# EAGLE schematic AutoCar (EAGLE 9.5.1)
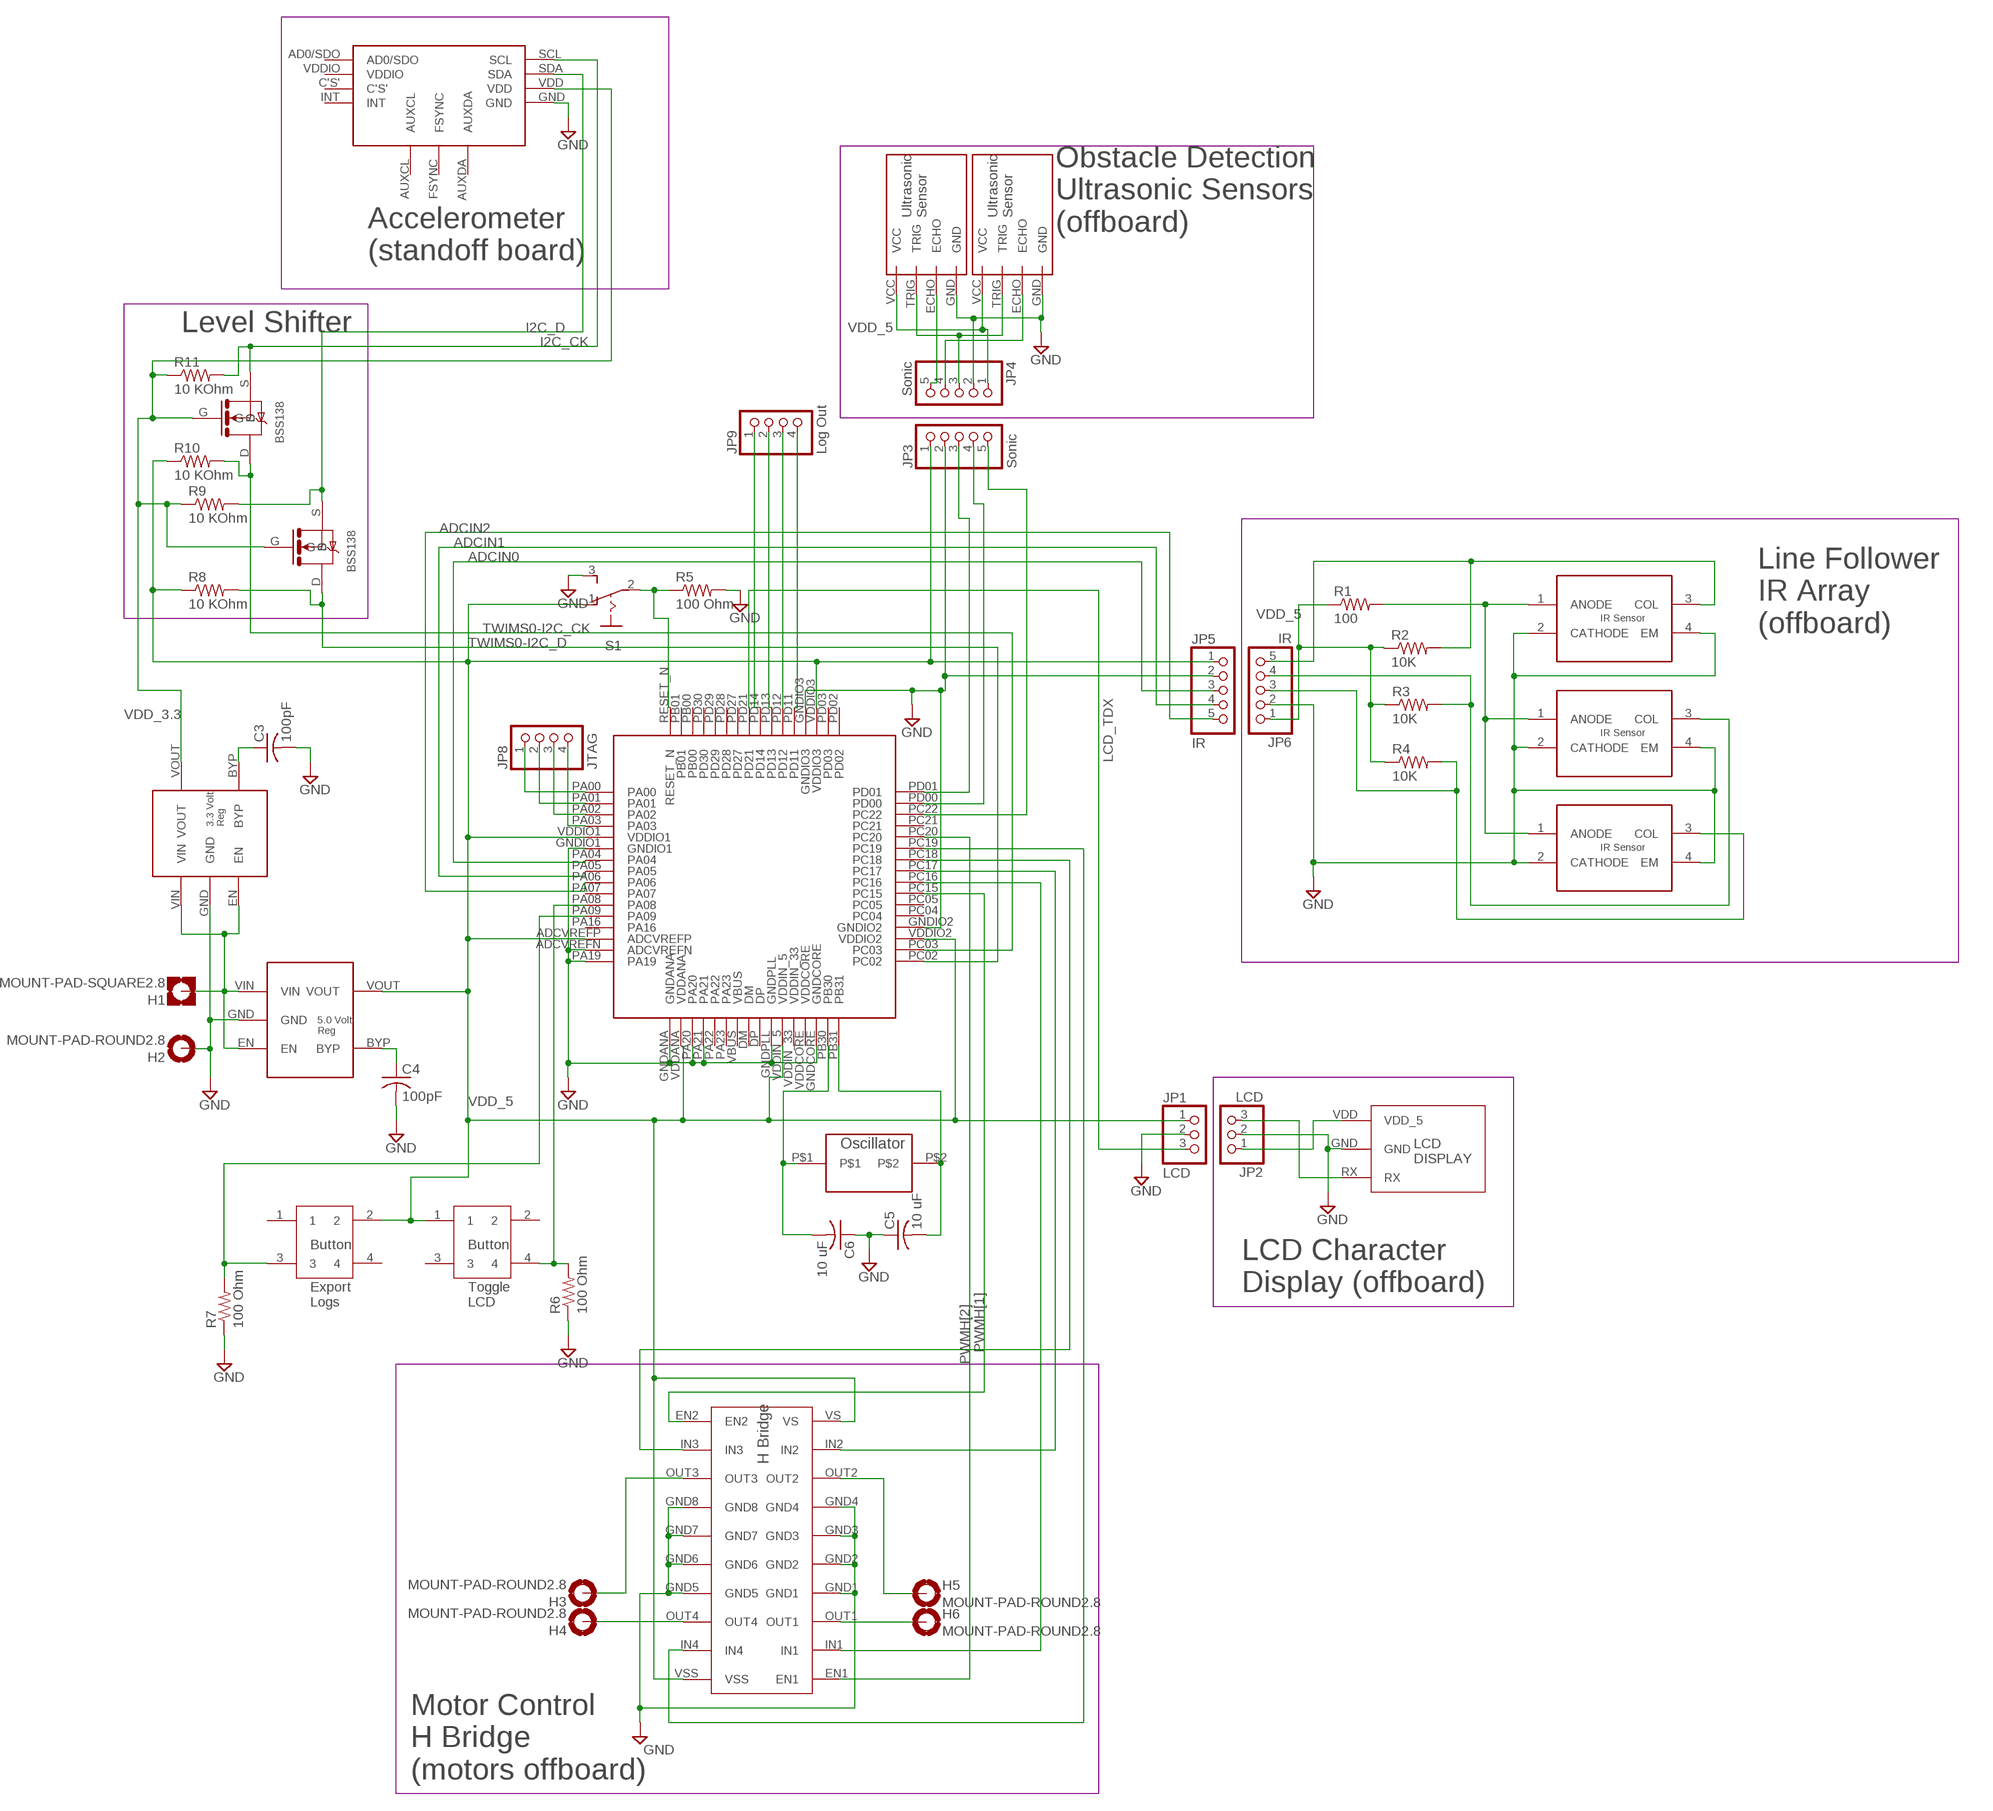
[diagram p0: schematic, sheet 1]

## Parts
C3  100pF  C-USC0805  [C0805]
C4  100pF  C-USC0805  [C0805]
C5  10 uF  C-USC0805  [C0805]
C6  10 uF  C-USC0805  [C0805]
H1  MOUNT-PAD-SQUARE2.8  [2,8-PAD-SQUARE]
H2  MOUNT-PAD-ROUND2.8  [2,8-PAD]
H3  MOUNT-PAD-ROUND2.8  [2,8-PAD]
H4  MOUNT-PAD-ROUND2.8  [2,8-PAD]
H5  MOUNT-PAD-ROUND2.8  [2,8-PAD]
H6  MOUNT-PAD-ROUND2.8  [2,8-PAD]
JP1  LCD  PINHD-1X3  [1X03]
JP2  LCD  PINHD-1X3  [1X03]
JP3  Sonic  PINHD-1X5  [1X05]
JP4  Sonic  PINHD-1X5  [1X05]
JP5  IR  PINHD-1X5  [1X05]
JP6  IR  PINHD-1X5  [1X05]
JP8  JTAG  PINHD-1X4  [1X04]
JP9  Log Out  PINHD-1X4  [1X04]
R1  100  R-US_M0805  [M0805]
R2  10K  R-US_M0805  [M0805]
R3  10K  R-US_M0805  [M0805]
R4  10K  R-US_M0805  [M0805]
R5  100 Ohm  R-US_M0805  [M0805]
R6  100 Ohm  R-US_M0805  [M0805]
R7  100 Ohm  R-US_M0805  [M0805]
R8  10 KOhm  R-US_M0805  [M0805]
R9  10 KOhm  R-US_M0805  [M0805]
R10  10 KOhm  R-US_M0805  [M0805]
R11  10 KOhm  R-US_M0805  [M0805]
S1  255SB  [255SB]
U$1  AT32UC3C2512C-A2UT  [TQFP-64]
U$2  QRE1113GR  [4-SMD]
U$3  QRE1113GR  [4-SMD]
U$4  QRE1113GR  [4-SMD]
U$5  SEN-15569  [HC-SR04]
U$6  SEN-15569  [HC-SR04]
U$7  AP2210K-5.0TRG1  [SC-74A]
U$8  SEN-13762  [MPU-9250]
U$10  AP2210K-3.3TRG1  [SC-74A]
U$11  ADAFRUIT-782  [LCD-3]
U$12  L293DD  [SOIC20]
U$14  LFXTAL003210BULK  [HC-49/US]
U$17  PTS645SM43SMTR92LFS  [SM43SMTR92LFS]
U$18  PTS645SM43SMTR92LFS  [SM43SMTR92LFS]
U$19  BSS138  [SOT23]
U$20  BSS138  [SOT23]

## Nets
ADCIN0: JP5.3 U$1.PA04
ADCIN1: JP5.4 U$1.PA05
ADCIN2: JP5.5 U$1.PA06
ECHO_L: JP3.5 JP4.5 U$1.PC22 U$6.ECHO
ECHO_R: JP3.4 JP4.4 U$1.PD00 U$5.ECHO
GND: C3.2 C4.2 C5.1 C6.1 H2.B2,8(MOUNT) JP1.2 JP2.2 JP3.2 JP4.2 JP5.2 JP6.2 R5.2 R6.1 R7.1 S1.3(S) U$1.ADCVREFN U$1.GNDANA U$1.GNDCORE U$1.GNDIO1 U$1.GNDIO2 U$1.GNDIO3 U$1.GNDPLL U$1.PA19 U$1.PA20 U$1.PA21 U$2.2(CATHODE) U$2.4(EM) U$3.2(CATHODE) U$3.4(EM) U$4.2(CATHODE) U$4.4(EM) U$5.GND U$6.GND U$7.GND U$8.GND U$10.GND U$11.GND U$12.GND1 U$12.GND2 U$12.GND3 U$12.GND4 U$12.GND5 U$12.GND6 U$12.GND7 U$12.GND8
I2C_CK: R11.2 U$8.SCL U$19.S
I2C_D: R9.2 U$8.SDA U$20.S
LCD_TDX: JP1.3 JP2.3 U$1.PD21 U$11.RX
N$1: JP2.1 U$11.VDD(VDD_5)
N$2: H3.B2,8(MOUNT) U$12.OUT3
N$3: H1.B2,8(MOUNT) U$7.EN U$7.VIN U$10.EN U$10.VIN
N$4: H4.B2,8(MOUNT) U$12.OUT4
N$5: H5.B2,8(MOUNT) U$12.OUT2
N$6: H6.B2,8(MOUNT) U$12.OUT1
N$7: JP9.4 U$1.PD11
N$8: C6.2 U$1.PB30 U$14.P$1
N$9: JP9.3 U$1.PD12
N$10: R5.1 S1.2(P) U$1.RESET_N
N$11: R6.2 U$1.PA08 U$18.4
N$12: R1.2 U$2.1(ANODE) U$3.1(ANODE) U$4.1(ANODE)
N$13: JP6.5 R2.2 U$2.3(COL)
N$14: C5.2 U$1.PB31 U$14.P$2
N$15: JP6.4 R3.2 U$3.3(COL)
N$16: JP6.3 R4.2 U$4.3(COL)
N$18: U$1.PC16 U$12.IN1
N$19: JP8.1 U$1.PA00
N$21: U$1.PC19 U$12.IN4
N$22: JP9.1 U$1.PD14
N$23: U$1.PC17 U$12.IN2
N$24: JP9.2 U$1.PD13
N$25: JP8.2 U$1.PA01
N$26: JP8.3 U$1.PA02
N$27: JP8.4 U$1.PA03
N$29: C3.1 U$10.BYP
N$30: C4.1 U$7.BYP
N$32: R7.2 U$1.PA09 U$17.3
N$33: U$1.PC18 U$12.IN3
PWMH[1]: U$1.PC15 U$12.EN2
PWMH[2]: U$1.PC20 U$12.EN1
TRIG: JP3.3 JP4.3 U$1.PD01 U$5.TRIG U$6.TRIG
TWIMS0-I2C_CK: R10.2 U$1.PC03 U$19.D
TWIMS0-I2C_D: R8.2 U$1.PC02 U$20.D
VDD_3.3: R9.1 R11.1 U$8.VDD U$10.VOUT U$19.G U$20.G
VDD_5: JP1.1 JP3.1 JP4.1 JP5.1 JP6.1 R1.1 R2.1 R3.1 R4.1 R8.1 R10.1 S1.1(O) U$1.ADCVREFP U$1.VDDANA U$1.VDDIN_5 U$1.VDDIO1 U$1.VDDIO2 U$1.VDDIO3 U$5.VCC U$6.VCC U$7.VOUT U$12.VS U$12.VSS U$17.2 U$18.1
Unconnected: U$1.DM U$1.DP U$1.PA07 U$1.PA16 U$1.PA22 U$1.PA23 U$1.PB00 U$1.PB01 U$1.PC04 U$1.PC05 U$1.PC21 U$1.PD02 U$1.PD03 U$1.PD27 U$1.PD28 U$1.PD29 U$1.PD30 U$1.VBUS U$1.VDDCORE U$1.VDDIN_33 U$8.AD0/SDO U$8.AUXCL U$8.AUXDA U$8.C'S' U$8.FSYNC U$8.INT U$8.VDDIO U$17.1 U$17.4 U$18.2 U$18.3

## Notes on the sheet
- Obstacle Detection
  Ultrasonic Sensors
  (offboard)
- Accelerometer
  (standoff board)
- Level Shifter
- Line Follower
  IR Array
  (offboard)
- LCD Character
  Display (offboard)
- Export
  Logs
- Toggle
  LCD
- Motor Control
  H Bridge
  (motors offboard)

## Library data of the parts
C3-C6 = rcl:C-US: CAPACITOR, American symbol; SPICEPREFIX: C
H1 = holes:MOUNT-PAD-SQUARE: MOUNTING PAD, square
H2-H6 = holes:MOUNT-PAD-ROUND: MOUNTING PAD, round
JP1 JP2 = pinhead:PINHD-1X3: PIN HEADER
JP3-JP6 = pinhead:PINHD-1X5: PIN HEADER
JP8 JP9 = pinhead:PINHD-1X4: PIN HEADER
R1-R11 = rcl:R-US_: RESISTOR, American symbol; SPICEPREFIX: R
S1 = switch:255SB: SLIDING SWITCH Distributor Buerklin, 11G810
U$1 = MILESTONE4LIB_E:AT32UC3C2512C-A2UT
U$2-U$4 = MILESTONE4LIB_E:QRE1113GR
U$5 U$6 = MILESTONE4LIB_E:SEN-15569
U$7 = MILESTONE4LIB_E:AP2210K-5.0TRG1
U$8 = miu:SEN-13762
U$10 = MILESTONE4LIB_E:AP2210K-3.3TRG1
U$11 = MILESTONE4LIB_E:ADAFRUIT-782
U$12 = MILESTONE4LIB_E:L293DD
U$14 = MILESTONE4LIB_E:LFXTAL003210BULK
U$17 U$18 = MILESTONE4LIB_E:PTS645SM43SMTR92LFS
U$19 U$20 = MILESTONE4LIB_E:BSS138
